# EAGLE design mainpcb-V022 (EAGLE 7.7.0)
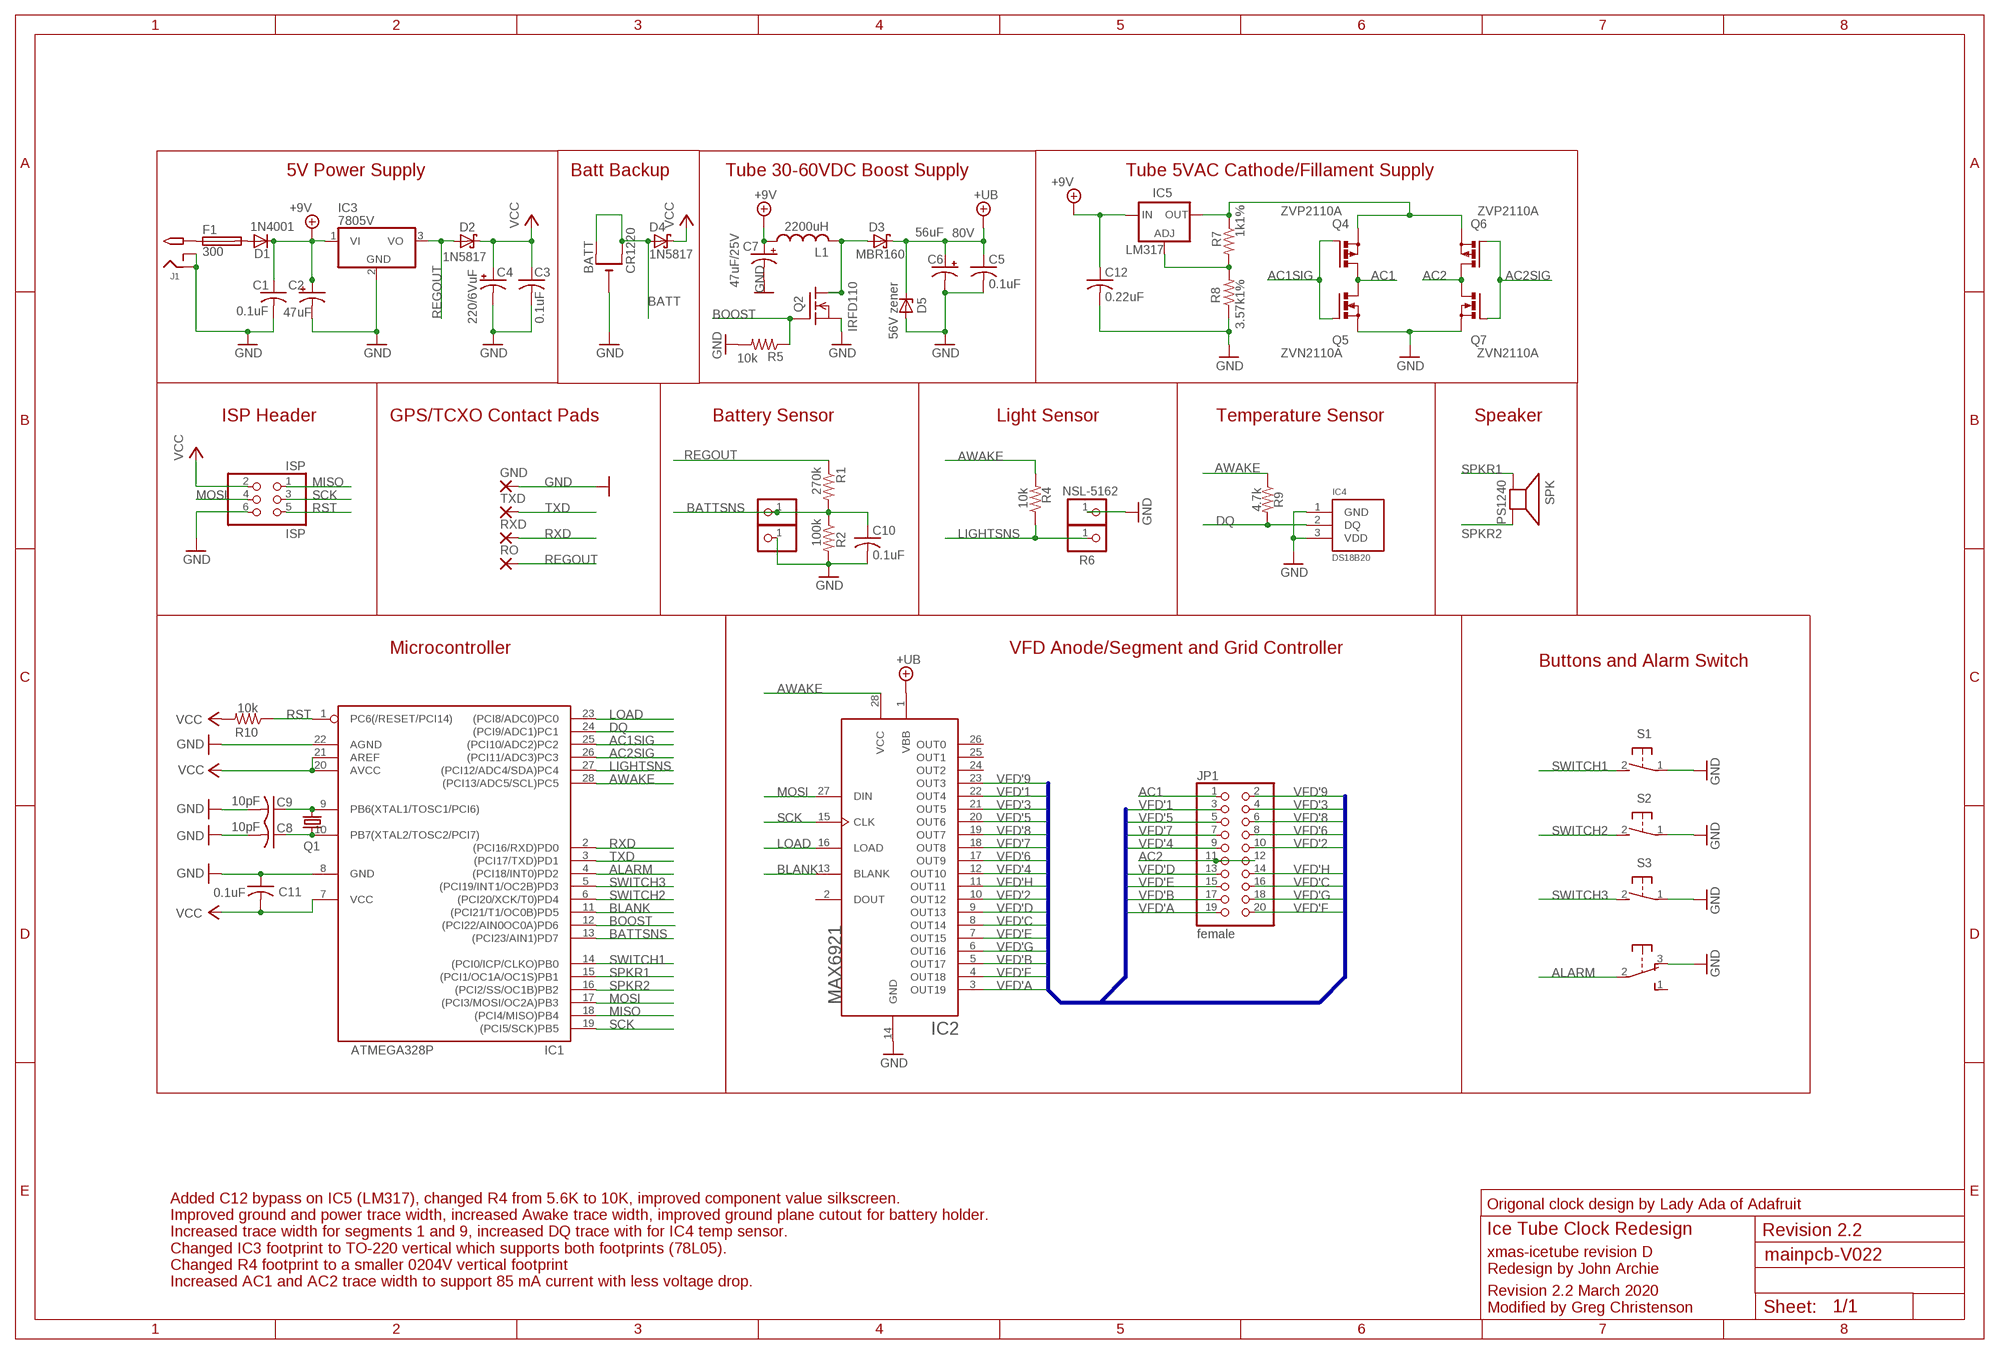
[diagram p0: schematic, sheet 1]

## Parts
BATT  CR1220  CR1220THM  [CR1220-THM]
C1  0.1uF  C-US025-025X050  [C025-025X050]
C2  47uF  CPOL-USE2.5-6  [E2,5-6]
C3  0.1uF  C-US025-025X050  [C025-025X050]
C4  220/6VuF  CPOL-USE2.5-6  [E2,5-6]
C5  0.1uF  C-US025-024X044  [C025-024X044]
C6  56uF  CPOL-USE3.5-8  [E3,5-8]
C7  47uF/25V  CPOL-USE2.5-6  [E2,5-6]
C8  10pF  C-US025-024X044  [C025-024X044]
C9  10pF  C-US025-024X044  [C025-024X044]
C10  0.1uF  C-US025-024X044  [C025-024X044]
C11  0.1uF  C-US025-025X050  [C025-025X050]
C12  0.22uF  C-US025-024X044  [C025-024X044]
CT2  PINHD-1X1  [1X01]
CT3  PINHD-1X1  [1X01]
D1  1N4001  1N4004  [DO41-10]
D2  1N5817  SCHOTTKY-DIODEDO41  [DO41-10]
D3  MBR160  SCHOTTKY-DIODEDO41  [DO41-10]
D4  1N5817  SCHOTTKY-DIODEDO41  [DO41-10]
D5  56V zener  ZENER-DIODEDO41Z10  [DO41Z10]
F1  300  FUSETE5  [TE5]
GND  1,6/0,9  [1,6/0,9]
IC1  ATMEGA328P  ATMEGA168PROUND  [DIL28/3]
IC2  MAX6921  [PLCC-S28]
IC3  7805V  7805TV  [TO220V]
IC4  DS18B20  [TO92]
IC5  LM317  [TO92-LINE]
ISP  ISP  PINHD-2X3  [2X03]
J1  2.1MMJACK  [PJ-102A]
JP1  female  PINHD-2X10  [2X10]
L1  2200uH  L  [6000]
Q1  32.768khz  CRYTALTC26V  [TC26V]
Q2  IRFD110  [DIL04]
Q4  ZVP2110A  [TO92-FLAT]
Q5  ZVN2110A  [TO92-FLAT]
Q6  ZVP2110A  [TO92-FLAT]
Q7  ZVN2110A  [TO92-FLAT]
R1  270k  R-US_0207/10  [0207/10]
R2  100k  R-US_0207/10  [0207/10]
R4  10k  R-US_0204/2V  [0204V]
R5  10k  R-US_0207/5V  [0207/5V]
R6  NSL-5162  PINHD-1X1  [1X01]
R6.1  PINHD-1X1  [1X01]
R7  1k1%  R-US_0207/5V  [0207/5V]
R8  3.57k1%  R-US_0207/5V  [0207/5V]
R9  4.7k  R-US_0207/10  [0207/10]
R10  10k  R-US_0207/5V  [0207/5V]
RO  1,6/0,9  [1,6/0,9]
RXD  1,6/0,9  [1,6/0,9]
S1  31-XX  [B3F-31XX]
S2  31-XX  [B3F-31XX]
S3  31-XX  [B3F-31XX]
SPK  PS1240  SPEAKER/PS12  [PS12]
SW1  OS102011MA1Q  [OS102011MA1Q]
TXD  1,6/0,9  [1,6/0,9]

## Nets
+9V: C1.1 C2.+ C7.+ C12.1 D1.C IC3.1(VI) IC5.3(IN) L1.1
+UB: C5.1 C6.+ D3.C D5.C IC2.1(VBB)
AC1: JP1.1 Q4.3(D) Q5.3(D)
AC1SIG: IC1.25((PCI10/ADC2)PC2) Q4.2(G) Q5.2(G)
AC2: JP1.11 JP1.12 Q6.3(D) Q7.3(D)
AC2SIG: IC1.26((PCI11/ADC3)PC3) Q6.2(G) Q7.2(G)
ALARM: IC1.4((PCI18/INT0)PD2) SW1.2(P)
AWAKE: IC1.28((PCI13/ADC5/SCL)PC5) IC2.28(VCC) R4.2 R9.1
BATT: BATT.+1(+) BATT.+2(+1) D4.A
BATTSNS: C10.1 CT2.1 IC1.13((PCI23/AIN1)PD7) R1.2 R2.1
BLANK: IC1.11((PCI21/T1/OC0B)PD5) IC2.13(BLANK)
BOOST: IC1.12((PCI22/AIN0OC0A)PD6) Q2.3(G) R5.1
DQ: IC1.24((PCI9/ADC1)PC1) IC4.2(DQ) R9.2
GND: BATT.- C1.2 C2.- C3.2 C4.- C5.2 C6.- C7.- C8.2 C9.2 C10.2 C11.1 C12.2 CT3.1 D5.A GND.1(P) IC1.8(GND) IC1.22(AGND) IC2.14(GND) IC3.2(GND) IC4.1(GND) IC4.3(VDD) ISP.6 J1.RING J1.RING_SW Q2.4(S) Q5.1(S) Q7.1(S) R2.2 R5.2 R6.1 R8.1 S1.1(P) S2.1(P) S3.1(P) SW1.3(O)
LIGHTSNS: IC1.27((PCI12/ADC4/SDA)PC4) R4.1 R6.1.1
LOAD: IC1.23((PCI8/ADC0)PC0) IC2.16(LOAD)
MISO: IC1.18((PCI4/MISO)PB4) ISP.1
MOSI: IC1.17((PCI3/MOSI/OC2A)PB3) IC2.27(DIN) ISP.4
N$1: C9.1 IC1.9(PB6(XTAL1/TOSC1/PCI6)) Q1.2
N$2: D3.A L1.2 Q2.1(D) Q2.2(D1)
N$3: C8.1 IC1.10(PB7(XTAL2/TOSC2/PCI7)) Q1.1
N$4: F1.1 J1.TIP
N$5: D1.A F1.2
N$6: IC5.1(ADJ) R7.2 R8.2
N$14: IC5.2(OUT) Q4.1(S) Q6.1(S) R7.1
REGOUT: D2.A IC3.3(VO) R1.1 RO.1(P)
RST: IC1.1(PC6(/RESET/PCI14)) ISP.5 R10.1
RXD: IC1.2((PCI16/RXD)PD0) RXD.1(P)
SCK: IC1.19((PCI5/SCK)PB5) IC2.15(CLK) ISP.3
SPKR1: IC1.15((PCI1/OC1A/OC1S)PB1) SPK.P$1(+)
SPKR2: IC1.16((PCI2/SS/OC1B)PB2) SPK.P$2(-)
SWITCH1: IC1.14((PCI0/ICP/CLKO)PB0) S1.2(S)
SWITCH2: IC1.6((PCI20/XCK/T0)PD4) S2.2(S)
SWITCH3: IC1.5((PCI19/INT1/OC2B)PD3) S3.2(S)
TXD: IC1.3((PCI17/TXD)PD1) TXD.1(P)
VCC: C3.1 C4.+ C11.2 D2.C D4.C IC1.7(VCC) IC1.20(AVCC) IC1.21(AREF) ISP.2 R10.2
VFD'1: IC2.22(OUT4) JP1.3
VFD'2: IC2.10(OUT12) JP1.10
VFD'3: IC2.21(OUT5) JP1.4
VFD'4: IC2.12(OUT10) JP1.9
VFD'5: IC2.20(OUT6) JP1.5
VFD'6: IC2.17(OUT9) JP1.8
VFD'7: IC2.18(OUT8) JP1.7
VFD'8: IC2.19(OUT7) JP1.6
VFD'9: IC2.23(OUT3) JP1.2
VFD'A: IC2.3(OUT19) JP1.19
VFD'B: IC2.5(OUT17) JP1.17
VFD'C: IC2.8(OUT14) JP1.16
VFD'D: IC2.9(OUT13) JP1.13
VFD'E: IC2.7(OUT15) JP1.15
VFD'F: IC2.4(OUT18) JP1.20
VFD'G: IC2.6(OUT16) JP1.18
VFD'H: IC2.11(OUT11) JP1.14
Unconnected: IC2.2(DOUT) IC2.24(OUT2) IC2.25(OUT1) IC2.26(OUT0) SW1.1(S) SW1.MT1(MT) SW1.MT2(MT)

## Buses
VFD'[1..9],VFD'_A,VFD'_B,VFD'_C,VFD'_D,VFD'_E,VFD'_F,VFD'_G,VFD'_H

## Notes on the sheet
- 5V Power Supply | Batt Backup | Tube 30-60VDC Boost Supply | Tube 5VAC Cathode/Fillament Supply
- 80V
- ISP Header | GPS/TCXO Contact Pads | Battery Sensor | Light Sensor | Temperature Sensor | Speaker
- Microcontroller | VFD Anode/Segment and Grid Controller
- Buttons and Alarm Switch
- Origonal clock design by Lady Ada of Adafruit
- Ice Tube Clock Redesign | Revision 2.2
- xmas-icetube revision D
- Redesign by John Archie
- Added C12 bypass on IC5 (LM317), changed R4 from 5.6K to 10K, improved component value silkscreen.
  Improved ground and power trace width, increased Awake trace width, improved ground plane cutout for battery holder.
  Increased trace width for segments 1 and 9, increased DQ trace with for IC4 temp sensor.
  Changed IC3 footprint to TO-220 vertical which supports both footprints (78L05).
  Changed R4 footprint to a smaller 0204V vertical footprint
  Increased AC1 and AC2 trace width to support 85 mA current with less voltage drop.
- Revision 2.2 March 2020
- Modified by Greg Christenson

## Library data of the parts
BATT = vfd:CR1220
C1 C3 C11 = minimidi:C-US: CAPACITOR, American symbol
C2 C4 C7 = minimidi:CPOL-US: POLARIZED CAPACITOR, American symbol
C5 C10 C12 = rcl-ez:C-US: CAPACITOR, American symbol
C6 = rcl-ez:CPOL-US: POLARIZED CAPACITOR, American symbol
C8 C9 = resistor:C-US: CAPACITOR, American symbol
CT2 CT3 R6 R6.1 = ybox2:PINHD-1X1: PIN HEADER
D1 = minimidi:1N4004: DIODE
D2-D4 = usbbuck:SCHOTTKY-DIODE: Schottky Diode
D5 = diode:ZENER-DIODE: Z-Diode
F1 = fuse:FUSE: Fuse
GND RO RXD TXD = wirepad:1,6/0,9: THROUGH-HOLE PAD
IC1 = avr:ATMEGA168*P: MICROCONTROLLER 16 kBytes FLASH 1 kBytes SRAM 512 Bytes EEPROM USART 8-channel 10 bit ADC
IC2 = vfd:MAX6921
IC3 = linear:78*: Positive VOLTAGE REGULATOR Source: http://cache.national.com/ds/LM/LM78L05.pdf http://www.fairchildsemi.com/ds/LM/LM7805.pdf
IC4 = jarchie:DS18B20
IC5 = jarchie:LM317: VOLTAGE REGULATOR
ISP = pinhead-ez:PINHD-2X3: PIN HEADER
J1 = minimidi:2.1MMJACK
JP1 = pinhead:PINHD-2X10: PIN HEADER
L1 = usbbuck:L
Q1 = crystal:CRYTAL: CRYSTAL
Q2 = vfd:IRFD110
Q4 Q6 = jarchie:ZVP2110A
Q5 Q7 = jarchie:ZVN2110A
R1 R2 R4 R5 R7-R10 = minimidi:R-US_: RESISTOR, American symbol
S1-S3 = switch-omron:31-XX: OMRON SWITCH
SPK = ybox2:SPEAKER: SPEAKER
SW1 = adaprog:OS102011MA1Q

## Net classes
0 default: clearance 0.205 mm

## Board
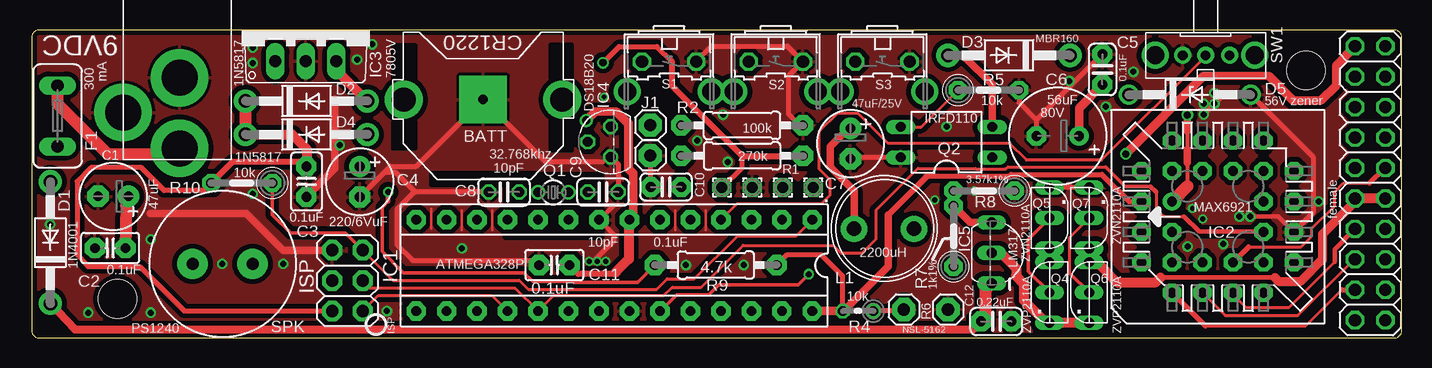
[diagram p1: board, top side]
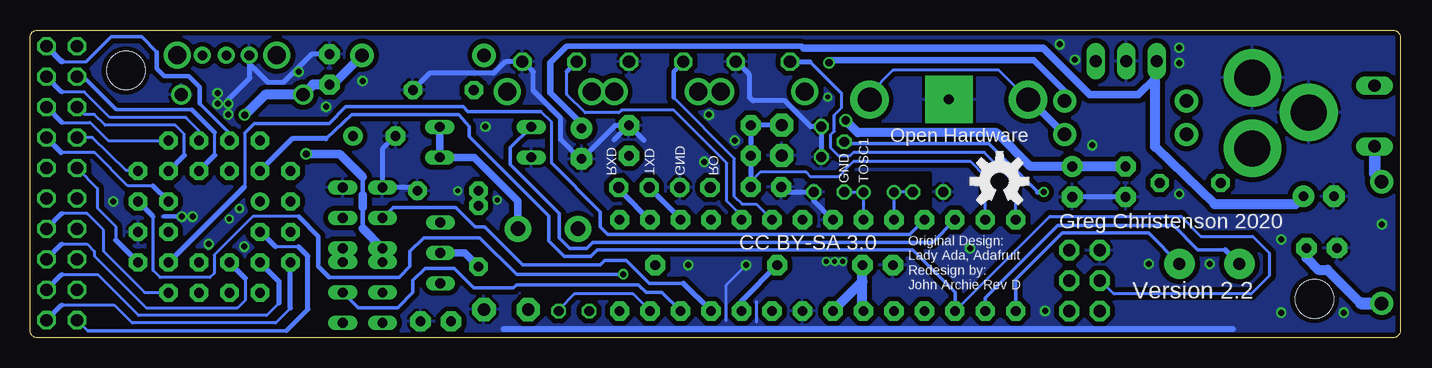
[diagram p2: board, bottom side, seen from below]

Size 114.2 x 25.71 mm. Coordinates in mm from the lower left corner, seen from the top.
Outline: 0,25.07 0,0.64 arc90 0.64,0 113.56,0 arc90 114.2,0.64 114.2,25.07 arc90 113.56,25.71 0.64,25.71 arc90 0,25.07
Copper layers (1*16): Top 0.0356mm / dielectric 1.5011mm / Bottom 0.0356mm
Design rules "LaenPCBOrder *": minimum track width 6mil, minimum drill 13mil, track to track 10mil, track to pad 10mil, pad to pad 10mil, via to via 10mil, smd to smd 6mil, copper to edge 15mil, drill to drill 8mil, minimum pad ring 7mil, minimum via ring 7mil, stop-mask expansion 4mil, vias tented up to drill 20mil, thermal gap 10mil
Holes 3.2 mm at 106.21,22.31 7.15,3.26

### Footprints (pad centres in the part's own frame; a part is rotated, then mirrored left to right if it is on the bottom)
CR1220-THM = drill 2 pad 3.175: +1 -6.604,0; +2 6.604,0 | drill 0.8 pad 3.962 square: - 0,0
C025-025X050 = drill 0.813 pad 1.676 octagon: 1 -1.27,0; 2 1.27,0
E2,5-6 = drill 0.813 pad 1.778: + -1.27,0 | drill 0.813 pad 1.778 octagon: - 1.27,0
C025-024X044 = drill 0.813 pad 1.676 octagon: 1 -1.27,0; 2 1.27,0
E3,5-8 = drill 0.813 pad 1.6: + -1.778,0 | drill 0.813 pad 1.6 octagon: - 1.778,0
C025-024X044' = drill 0.813 octagon: 1 -1.27,0; 2 1.27,0
1X01 = drill 1.016 pad 1.93 octagon: 1 0,0
DO41-10 = drill 1.118 pad 1.93: A 5.08,0; C -5.08,0
DO41Z10 = drill 1.118: A 5.08,0; C -5.08,0
TE5 = drill 1.016 long: 1 -2.54,0; 2 2.54,0
1,6/0,9 = drill 0.914 pad 1.6 octagon: 1 0,0
DIL28/3 = drill 0.813 pad 1.6 octagon: 1 -16.51,-3.81; 2 -13.97,-3.81; 3 -11.43,-3.81; 4 -8.89,-3.81; 5 -6.35,-3.81; 6 -3.81,-3.81; 7 -1.27,-3.81; 8 1.27,-3.81; 9 3.81,-3.81; 10 6.35,-3.81; 11 8.89,-3.81; 12 11.43,-3.81; 13 13.97,-3.81; 14 16.51,-3.81; 15 16.51,3.81; 16 13.97,3.81; 17 11.43,3.81; 18 8.89,3.81; 19 6.35,3.81; 20 3.81,3.81; 21 1.27,3.81; 22 -1.27,3.81; 23 -3.81,3.81; 24 -6.35,3.81; 25 -8.89,3.81; 26 -11.43,3.81; 27 -13.97,3.81; 28 -16.51,3.81
PLCC-S28 = drill 0.813 pad 1.524: 1 1.27,3.81 | drill 0.813 pad 1.524 octagon: 2 -1.27,6.35; 3 -1.27,3.81; 4 -3.81,6.35; 5 -6.35,3.81; 6 -3.81,3.81; 7 -6.35,1.27; 8 -3.81,1.27; 9 -6.35,-1.27; 10 -3.81,-1.27; 11 -6.35,-3.81; 12 -3.81,-6.35; 13 -3.81,-3.81; 14 -1.27,-6.35; 15 -1.27,-3.81; 16 1.27,-6.35; 17 1.27,-3.81; 18 3.81,-6.35; 19 6.35,-3.81; 20 3.81,-3.81; 21 6.35,-1.27; 22 3.81,-1.27; 23 6.35,1.27; 24 3.81,1.27; 25 6.35,3.81; 26 3.81,6.35; 27 3.81,3.81; 28 1.27,6.35
TO220V = drill 1.016 long: 1 -2.54,-2.54; 2 0,-2.54; 3 2.54,-2.54
TO92 = drill 0.813 octagon: 1 1.27,0; 2 0,1.905; 3 -1.27,0
TO92-LINE = drill 0.813 long: 1 -2.54,0; 2 0,0; 3 2.54,0
2X03 = drill 1.016 pad 1.676 octagon: 1 -2.54,-1.27; 2 -2.54,1.27; 3 0,-1.27; 4 0,1.27; 5 2.54,-1.27; 6 2.54,1.27
PJ-102A = drill 3 pad 4.8: RING 0.1,-3.39; RING_SW -4.6,-6.29; TIP 0.1,-9.29
2X10 = drill 1.016 octagon: 1 -11.43,-1.27; 2 -11.43,1.27; 3 -8.89,-1.27; 4 -8.89,1.27; 5 -6.35,-1.27; 6 -6.35,1.27; 7 -3.81,-1.27; 8 -3.81,1.27; 9 -1.27,-1.27; 10 -1.27,1.27; 11 1.27,-1.27; 12 1.27,1.27; 13 3.81,-1.27; 14 3.81,1.27; 15 6.35,-1.27; 16 6.35,1.27; 17 8.89,-1.27; 18 8.89,1.27; 19 11.43,-1.27; 20 11.43,1.27
6000 = drill 1.2 pad 2.184: 1 -2.5,0; 2 2.5,0
TC26V = drill 0.813: 1 -1.27,0; 2 1.27,0
DIL04 = drill 0.813 long: 1 -1.27,-3.81; 2 1.27,-3.81; 3 1.27,3.81; 4 -1.27,3.81
TO92-FLAT = drill 0.813 long: 1 -2.54,0; 2 0,0; 3 2.54,0
0207/10 = drill 0.813 pad 1.676 octagon: 1 -5.08,0; 2 5.08,0
0204V = drill 0.813 octagon: 1 -1.27,0; 2 1.27,0
0207/5V = drill 0.813 pad 1.524 octagon: 1 -2.54,0; 2 2.54,0
B3F-31XX = drill 1.016 octagon: 1 -2.261,-1.245; 2 2.261,-1.245 | drill 1.499 pad 2.159: 3 -3.505,1.245; 4 3.505,1.245
PS12 = drill 1 pad 2.54: P$1 -2.5,0; P$2 2.5,0
OS102011MA1Q = drill 0.8 pad 1.422: 1 -2,0; 2 0,0; 3 1.9,0 | drill 1.5 pad 2.184: MT1 -4.1,0; MT2 4.2,0

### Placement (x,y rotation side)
BATT  37.63,19.9 0 top
C1  6.55,7.51 180 top
C2  6.81,11.82 180 top
C3  22.9,13.04 270 top
C4  27.35,13.04 270 top
C5  89.24,22.41 90 top
C6  85.51,16.85 180 top
C7  68.24,16.22 270 top
C8  10pF  [C025-024X044']  39.36,12.18 180 top
C9  10pF  [C025-024X044']  47.62,12.18 0 top
C10  52.87,12.6 180 top
C11  43.56,6.08 0 top
C12  80.39,1.38 0 top
CT2  51.56,17.77 0 top
CT3  51.56,15.23 0 top
D1  1.57,7.96 90 top
D2  22.9,19.77 0 top
D3  81.45,23.58 180 top
D4  22.9,16.98 0 top
D5  96.52,20.31 0 top
F1  2.15,18.53 270 top
GND  60.07,12.56 0 top
IC1  48.56,6.06 180 top
IC2  98.85,10.12 90 top
IC3  22.86,25.64 0 top
IC4  48.25,16.37 90 top
IC5  80.01,7.1 270 top
ISP  26.33,4.79 90 top
J1  12.23,25.11 0 top
JP1  111.55,12.92 270 top
L1  71.04,9.11 0 top
Q1  43.48,12.15 0 top
Q2  76.24,16.35 90 top
Q4  84.83,3.8 90 top
Q5  84.83,10.02 270 top
Q6  88.13,3.8 90 top
Q7  88.13,10.02 270 top
R1  59.21,15.2 180 top
R2  59.21,17.74 0 top
R4  68.88,2.25 180 top
R5  79.75,20.69 0 top
R6  76.37,2.38 0 top
R6.1  72.69,2.38 0 top
R7  76.83,8.5 90 top
R8  79.37,12.28 180 top
R9  57.02,6.08 180 top
R10  17.52,12.94 180 top
RO  57.53,12.56 0 top
RXD  65.15,12.56 0 top
S1  53.13,21.81 180 top
S2  62.02,21.81 180 top
S3  70.91,21.81 180 top
SPK  15.92,6.19 180 top
SW1  97.83,23.58 180 top
TXD  62.61,12.56 0 top
U$1  [OSHW-LOGO-M]  33.4,13.07 0 bottom

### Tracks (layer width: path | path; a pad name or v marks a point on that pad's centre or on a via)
+9V
  Top 0.406: 68.04,17.49 C7.+
  Top 0.61: L1.1 68.54,12.27 66.54,14.26 66.54,15.99 68.04,17.49
  Top 0.686: D1.C 3.6,0.72 78.46,0.72 C12.1
  Top 0.813: C12.1 79.12,1.51
  Top 1.016: C2.+ 8.08,11.24 7.87,11.04 C1.1 | 79.12,1.51 79.5,1.89 79.5,4.05 IC5.3
  Bottom 0.406: 49.7,24.17 49.88,24.35 | 20.36,15.91 20.44,15.96 | IC3.1 20.44,23.1 20.44,22.85
  Bottom 0.457: 49.88,24.35 69.49,24.35 70.86,22.97
  Bottom 0.559: 70.86,22.97 70.86,20.49 68.24,17.87
  Bottom 0.61: 49.7,24.17 29.76,24.17 25.9,20.31 21.84,20.31 20.44,21.7 | 68.24,17.87 C7.+
  Bottom 0.711: 15.49,11.16 20.36,15.91
  Bottom 0.813: 20.44,15.96 20.44,21.7 20.44,22.85 | 15.49,11.16 8.74,11.16 C2.+ | C1.1 7.82,6.67 6.85,5.7 6.09,5.7 3.3,2.91 | 1.59,2.91 D1.C
  Bottom 1.016: 1.52,2.93 D1.C | 3.3,2.91 1.59,2.91
+UB  (via drill 0.6)
  Top 0.33: 96.31,17.26 96.31,15.71 | 96.31,14.64 96.31,12.67
  Top 0.61: v96.31,18.61 96.31,17.26 | 96.31,15.71 96.31,14.64
  Top 0.711: C5.1 87.29,19.2 C6.+
  Top 1.016: 96.31,12.67 IC2.1
  Bottom 0.406: 88.97,21.14 C5.1
  Bottom 0.711: D3.C 88.97,21.14
  Bottom 0.813: C5.1 90.6,21.14 D5.C 94.61,20.31 v96.31,18.61
AC1  (via drill 0.6)
  Top 0.508: JP1.1 110.28,24.29
  Top 0.61: Q4.3 Q5.3
  Top 0.686: 103.12,21.83 97.66,21.83
  Top 0.711: 110.28,24.29 108.71,22.72 108.71,21.07 107.44,19.8 105.15,19.8 103.12,21.83 | 97.66,21.83 v91.18,15.35
  Bottom 0.356: 86.48,13.45 86.48,11.93 | 86.48,10.91 86.48,9.13
  Bottom 0.711: v91.18,15.35 88.39,15.35 86.48,13.45 | 86.48,11.93 86.48,10.91 | 86.48,9.13 Q5.3
AC1SIG
  Top 0.305: Q5.2 83.05,8.24 83.05,5.58 Q4.2
  Bottom 0.305: Q5.2 83.94,10.91 78.73,10.91 77.08,9.26 76.32,9.26 73.15,6.08 66.67,6.08 66.29,6.46 64.51,6.46 62.61,4.56 59.76,4.56
  Bottom 0.406: IC1.25 59.76,4.56
AC2
  Top 0.381: 94.08,5.04 103.6,5.04
  Top 0.61: JP1.11 110.28,11.36 | Q7.3 Q6.3 88.77,6.34
  Top 0.762: 110.28,11.36 107.56,8.65 107.56,6.54 105.76,4.74 103.91,4.74 103.6,5.04
  Top 0.813: JP1.12 JP1.11 | 94.08,5.04 93.7,4.66 90.44,4.66 88.77,6.34
AC2SIG
  Top 0.254: Q7.2 86.48,8.37 86.48,5.45
  Top 0.305: 86.48,5.45 Q6.2
  Bottom 0.305: IC1.26 61.53,3.8 62.86,3.8 63.49,4.43 73.66,4.43 73.91,4.18 77.21,4.18 78.86,5.83 81.28,5.83 82.29,4.81 82.29,3.8 83.56,2.53 86.86,2.53 Q6.2
ALARM
  Top 0.254: IC1.4 58.79,11.21 65.83,11.21 66.54,11.93 66.54,13.2 65.65,14.08 65.65,17.26 67.18,18.78 68.83,18.78 71.37,16.24 81.53,16.24 82.93,14.85 89.15,14.85 97.83,23.53 SW1.2
AWAKE
  Top 0.254: 67.6,2.34 67.56,2.3 R4.2 | 74.54,13.45 74.62,13.5
  Top 0.406: IC2.28 91.46,11.39 89.2,13.65 81.63,13.65 81.45,13.5 74.62,13.5 | 67.56,2.3 67.56,5.19 65.78,6.97 62.99,6.97 R9.1 | 67.6,2.34 67.62,2.21
  Top 0.508: 71.37,10.27 74.54,13.45
  Top 0.61: 71.37,10.27 71.37,5.96 67.62,2.21
  Top 0.711: IC1.28 R4.2
BATT
  Bottom 0.254: BATT.+1 33.47,22.34 42.29,22.34 44.24,20.39
  Bottom 0.406: 30.9,19.9 BATT.+1 | BATT.+2 44.24,20.39 44.24,20.61
  Bottom 0.61: D4.A 30.9,19.9
BATTSNS
  Bottom 0.254: IC1.13 34.59,13.5 35.81,14.72 45.59,14.72 46.86,13.45 49.14,13.45 49.52,13.83 53.37,13.83 54.13,13.07 54.13,12.65
  Bottom 0.406: CT2.1 54.1,17.77 R2.1 R1.2 54.13,12.65 C10.1
BLANK
  Bottom 0.254: 96.31,17.08 96.31,12.64 | 39.67,9.85 IC1.11 | IC2.13 102.64,6.31 | 70.73,14.59 70.73,18.02 71.62,18.91 71.75,18.91
  Bottom 0.305: 96.31,17.08 95.5,17.89 89.28,17.89 87.88,19.29 78.1,19.29 77.72,18.91 71.75,18.91 | 39.67,9.85 40.89,8.62 66.04,8.62 66.67,9.26 66.67,10.53 70.73,14.59
  Bottom 0.406: 102.64,6.31 96.31,12.64
BOOST
  Top 0.254: Q2.3 74.14,17.62 R5.1
  Bottom 0.254: 37.13,9.85 IC1.12
  Bottom 0.305: Q2.3 74.16,15.88 74.16,14.47 70.1,10.4 70.1,8.37 69.21,7.48 67.81,7.48 67.31,7.99 38.98,7.99 37.13,9.85
DQ  (via drill 0.5)
  Top 0.305: R9.2 50.52,4.66 45.21,4.66 45.13,4.74 41.75,4.74 41.02,5.45 30.98,5.45 29.21,7.23 29.21,10.91 29.71,11.42
  Top 0.406: 29.71,11.42 v29.71,12.18
  Bottom 0.254: 46.1,16.37 IC4.2 45.97,16.24
  Bottom 0.305: 30.22,12.18 34.28,16.24 45.97,16.24
  Bottom 0.406: R9.2 54.91,3.12 IC1.24 | 30.22,12.18 v29.71,12.18
GND  (via drill 0.4, 0.5)
  Top 0.203: 53.64,10.66 53.64,9 | 56.18,10.66 56.18,9 | 33.32,10.78 33.32,9.13 | 35.86,10.66 35.86,9 | 38.4,10.66 38.4,9
  Top 0.356: IC1.8 48.51,8.65 | IC2.14 105.18,8.85 103.91,10.12 v101.54,10.12 | 47.26,9.81 48.49,11.04
  Top 0.406: IC2.14 106.8,10.46 106.8,15.1 D5.A 99.34,20.31 v97.69,18.66 | 37.53,19.8 BATT.- | BATT.- 42.82,14.72 47.62,14.72 IC4.3 48.89,14.47 C9.2 | 12.35,21.7 J1.RING | BATT.- 32.05,14.31 29.89,14.31 29.37,13.79 | C8.2 31.97,12.18 31.92,12.23 | C5.2 83.73,18.18 | R5.2 82.29,19.63 83.73,18.18 | CT3.1 51.56,12.62 C10.2 | S1.1 55.39,23.12 56.64,24.37 62.99,24.37 64.28,23.08 S2.1 63.11,21.89 63.11,18.66 64,17.77 64.26,17.77 R2.2 | C4.- 29.37,13.79 | 31.92,12.23 30.36,13.79 29.37,13.79 | C11.1 41.9,6.46 31.75,6.46 30.48,7.73 30.48,10.78 31.92,12.23 | 48.51,8.65 48.51,8.12 46.79,6.4 v46.46,6.4 | Q2.4 68.37,15.08 C7.- | 83.73,18.18 C6.- | Q7.1 Q5.1
  Top 0.61: ISP.6 20.98,7.33 17.9,10.4 9.9,10.4 | C3.2 25.27,14.14 25.27,19.93
  Bottom 0.254: 56.18,1.46 56.18,4.43 v54.53,6.08 | 53.64,1.33 53.64,3.04
  Bottom 0.356: 101.93,10.12 103.04,10.12
  Bottom 0.406: IC4.3 IC4.1 49.14,17.64 51.3,19.8 53.97,19.8 54.22,20.05 54.22,21.96 55.32,23.05 S1.1 | C5.2 90.73,23.68 93.09,21.32 94.36,21.32 95.93,22.9 SW1.3 95.88,23.53 95.88,21.7 97.69,19.9 v97.69,18.66 | 73.15,23.03 S3.1 | S3.1 74.59,23.05 75.56,22.09 80.89,22.09 R5.2 | J1.RING_SW 9.43,18.82 | IC1.8 48.89,11.47 C9.2 51.25,12.18 C10.2 | 63.04,16.5 R2.2 65.45,17.74 C7.- 68.37,14.95 69.97,16.55 69.97,18.35 72.26,20.64 72.26,22.21 73.1,23.05 S3.1 | C3.2 C4.- | C6.- 84.83,15.76 Q5.1 81.91,12.56 R8.1 | 64.28,17.79 65.53,16.55
  Bottom 0.508: 74.74,0.75 13.96,0.75
  other vias: 47.84,6.4 97.68,19.55 98.57,19.55 98.57,20.43 89.53,19.29 86.48,21.45 76.25,17.64 97.61,9.94 99.31,7.84 96.34,7.63 96.74,10.81 100.66,10.12 59.35,6.08 35.86,7.48 1.54,9.49 9.93,2.12 29.61,2.25 15.9,6.19 9.93,8.22 18.44,12.03 4.72,2.12 20.98,6.19 25.67,16.09 18.44,24.22 18.44,22.95 107.26,11.39 47.15,6.4 27.12,23.23 28.39,24.5 47.71,20.12 91.82,22.21 75.26,11.52 78.56,12.28 58.01,14.69 55.47,16.47 57.63,18.63
  pour Bottom (isolate 0.406, rank 2): -0.01,25.64 -0.01,-0.01 114.17,-0.01 114.17,25.64
  pour Top (isolate 0.406, rank 2): -0.01,25.64 -0.01,-0.01 114.17,-0.01 114.17,25.64
LIGHTSNS
  Top 0.406: R6.1.1 73.5,2.38 73.4,2.27 72.71,2.27 R4.1
  Bottom 0.254: IC1.27 63.95,3.67 68.83,3.67 70.15,2.35
  Bottom 0.406: 70.15,2.35 R4.1
LOAD  (via drill 0.5)
  Top 0.254: 52.42,2.25 IC1.23
  Top 0.305: 52.42,2.25 53.78,3.61 56.45,3.61 57.27,4.43 63.88,4.43 v64.77,5.32
  Bottom 0.254: 91.82,10.15 95.63,10.15 98.85,6.92 98.85,5.4 99.21,5.04 103.35,5.04 103.93,5.63 103.93,10.13
  Bottom 0.305: v64.77,5.32 73.66,5.32 76.7,8.37 81.4,8.37 82.55,7.23 82.55,5.96 83.43,5.07 89.28,5.07
  Bottom 0.356: 91.82,10.15 90.17,8.5 90.17,5.96 89.28,5.07
  Bottom 0.406: 103.93,10.13 IC2.16
MISO
  Top 0.254: IC1.18 39.64,2.25 38.35,3.54 28.9,3.54 ISP.1
MOSI
  Bottom 0.254: ISP.4 24.99,4.79 23.87,3.67 12.44,3.67 10.92,5.19 10.92,7.1 12.31,8.5 16.63,8.5 18.28,10.15 29.21,10.15 37.1,2.25 IC1.17 37.1,2.52
  Bottom 0.305: 89.53,16.62 87.37,18.66 78.48,18.66 77.59,17.64 77.59,16.8 70.99,10.2 70.99,8.12 69.67,6.79 67.48,6.79 66.92,7.35 40.63,7.35 37.1,3.82 37.1,2.52
  Bottom 0.406: 89.53,16.62 92.35,16.62 IC2.27
N$1
  Bottom 0.254: IC1.9 Q1.2 44.77,12.18 C9.1
N$2
  Top 0.406: 77.62,23.58 77.72,23.48
  Top 0.61: D3.A 77.62,23.58 | 77.72,23.48 80.05,21.17 Q2.2
  Bottom 0.406: 80.03,15.1 Q2.1
  Bottom 0.61: Q2.2 Q2.1 77.19,15.08 73.54,11.42 L1.2
N$3
  Bottom 0.254: IC1.10 Q1.1 42.18,12.18 C8.1
N$4
  Top 0.813: 11.87,15.35 J1.TIP
  Top 1.016: F1.1 2.15,19.55 6.34,15.35 11.87,15.35
N$5
  Bottom 0.965: F1.2 2.15,13.73 D1.A
N$6
  Top 0.61: R7.2 78.23,9.64 IC5.1
  Bottom 0.61: R8.2 R7.2
N$9
  cutout Top: 30.09,24.5 32,24.5 32,15.74 30.09,15.74
N$14
  Top 0.61: 84.2,1.64 84.58,1.51 Q4.1
  Top 0.813: Q6.1 Q4.1 | IC5.2 80.77,7.1 82.04,5.83 82.04,5.19 82.7,4.53 82.7,3.14 84.2,1.64
  Bottom 0.61: R7.1 77.97,7.1 IC5.2
N$18
  cutout Bottom: 39.24,8.24 39.24,13.7 47.75,13.7 47.75,8.24
N$19
  cutout Top: 39.49,13.7 47.49,13.7 47.49,8.37 39.49,8.37
N$21
  cutout Top: 33.27,13.83 42.29,13.83 42.29,12.69 33.27,12.69
N$23
  cutout Top: 43.17,24.5 43.17,15.61 45.08,15.61 45.08,24.5
REGOUT  (via drill 0.6)
  Top 0.406: v47.62,22.97 48.97,24.32 52.12,24.32 53.34,23.1 | RO.1 59.2,14.24 59.2,15.2
  Top 0.508: R1.1 59.2,15.2 53.34,21.07 53.34,23.1
  Top 0.813: D2.A 25.39,22.36 IC3.3
  Bottom 0.559: D2.A 27.98,20.61 30.55,23.18 47.42,23.18 v47.62,22.97
RST
  Top 0.254: IC1.1 63.69,8.5 58.8,8.5 55.24,4.94 52.95,4.94 52.09,4.08 41.37,4.08 40.63,4.81 30.12,4.81 ISP.5 27.58,7.33
  Top 0.305: 27.58,7.33 26.16,8.75 21.59,8.75 20.06,10.27 R10.1
RXD
  Bottom 0.305: IC1.2 62.58,9.87 | 64.77,12.05 RXD.1
  Bottom 0.406: 62.58,9.87 64.77,12.05
SCK
  Top 0.254: 93.72,12.18 93.72,10.78 94.36,10.15 96.03,10.15 | ISP.3 28.21,4.18 40.28,4.18 IC1.19 43.5,3.54 52.7,3.54 53.4,4.24 55.81,4.24 59.3,7.73 66.8,7.73 67.43,7.1 69.21,7.1 70.35,8.24 70.35,10.66 73.86,14.16 78.66,14.16 78.73,14.08 81.17,14.08 81.38,14.29 89.53,14.29 | 102.61,8.88 IC2.15
  Top 0.305: 93.24,12.66 91.16,12.66 89.53,14.29
  Top 0.356: 93.24,12.66 93.72,12.18 | 96.03,10.15 97.3,8.88 102.61,8.88
SPKR1
  Bottom 0.305: IC1.15 32.05,4.89 28.19,8.75 20.98,8.75 SPK.P$1
SPKR2
  Bottom 0.305: IC1.16 34.59,3.37 28.57,9.39 18.9,9.39 16.87,7.35 14.6,7.35
  Bottom 0.406: SPK.P$2 14.6,7.35
SWITCH1
  Bottom 0.254: IC1.14 32.05,12.86 34.67,15.48 45.59,15.48 45.87,15.2 46.81,15.2 47.49,15.89 47.49,16.93 47.16,17.26 47.16,18.58 46.6,19.16 46.6,20.43
  Bottom 0.305: 49.22,23.05 46.6,20.43
  Bottom 0.406: S1.2 49.22,23.05
SWITCH2
  Bottom 0.254: IC1.6 53.66,11.16 54.86,11.16 55.49,11.8 55.49,14.97 60.57,20.05
  Bottom 0.356: 60.57,20.05 60.57,22.23 S2.2
SWITCH3
  Bottom 0.254: IC1.5 54.91,10.19 56.13,11.42 56.13,14.59 60.57,19.04 64.89,19.04 65.14,18.79 67.93,18.79 69.46,20.32 69.46,22.23
  Bottom 0.356: S3.2 69.46,22.23
TXD
  Bottom 0.305: IC1.3 60.17,10.12 | 62.48,12.43 TXD.1
  Bottom 0.406: 60.17,10.12 62.48,12.43
VCC  (via drill 0.7)
  Top 0.406: ISP.2 12.72,2.25 9.01,5.96 4.69,5.96 3.81,6.97 3.81,13.07 4.95,14.21 9.14,14.21 11.04,12.31 14.35,12.31 R10.2 | C3.1 22.9,14.33 | 49.78,9.89 49.8,9.87 IC1.7
  Top 0.508: C11.2 45.56,5.35 48.53,5.35 48.69,5.5 | R10.2 16.75,14.71 22.52,14.71 22.9,14.33
  Top 0.711: 50.13,13.73 50.13,10.23 IC1.7 | v46.22,18.15 46.98,18.91 48.71,18.91 49.73,17.89
  Top 0.762: 49.73,17.89 49.73,14.14 50.13,13.73
  Top 0.813: 49.78,9.89 49.78,6.59 48.69,5.5 | D4.C 21.71,16.98 22.92,15.77 C3.1
  Top 1.016: D2.C D4.C
  Bottom 0.406: IC1.20 44.83,2.33
  Bottom 0.711: 44.83,4.71 C11.2
  Bottom 0.762: v46.22,18.15 45.21,17.13 33.65,17.13 30.83,14.31 C4.+
  Bottom 0.813: C3.1 C4.+ | 44.83,2.33 C11.2 | IC1.21 44.83,4.71
VFD'1
  Bottom 0.254: 110.21,21.81 JP1.3 | 98.8,15.25 98.8,17.13
  Bottom 0.305: 100.73,19.06 107.01,19.06
  Bottom 0.33: 107.01,19.06 109.75,21.81
  Bottom 0.356: 98.8,17.13 100.73,19.06
  Bottom 0.406: 109.75,21.81 JP1.3 | IC2.22 98.8,15.25
VFD'2
  Top 0.254: 101.41,7.61 105.79,7.61 106.68,8.5 106.68,9.13 108.58,11.04 108.58,12.18 109.32,12.92 111.48,12.92 | 112.75,14.19 JP1.10
  Top 0.406: IC2.10 101.41,7.61 | 111.48,12.92 112.75,14.19
VFD'3
  Bottom 0.254: IC2.21 100.12,17.31 101.21,18.4 107.54,18.4 109.67,20.54 111.55,20.54
  Bottom 0.406: 111.55,20.54 JP1.4
VFD'4
  Bottom 0.254: JP1.9 108.58,12.49 108.58,10.83 107.06,9.31 107.06,8.17
  Bottom 0.406: 107.06,8.17 IC2.12
VFD'5
  Bottom 0.254: IC2.20 102.66,13.91 | 101.34,15.23 101.34,17.01 102.1,17.77 107.95,17.77 108.83,18.66 109.67,18.66 JP1.5
  Bottom 0.406: 102.66,13.91 101.34,15.23
VFD'6
  Bottom 0.254: 103.95,12.69 106.04,12.69 108.81,15.46 111.6,15.46 | 112.82,16.67 JP1.8
  Bottom 0.406: IC2.17 103.95,12.69 | 111.6,15.46 112.82,16.67
VFD'7
  Bottom 0.254: IC2.18 105.22,13.96 106.17,13.96 109.01,16.73 JP1.7
VFD'8
  Bottom 0.254: 111.55,18 109.19,18 107.67,16.47 IC2.19
  Bottom 0.406: JP1.6 111.55,18
VFD'9
  Bottom 0.254: 111.55,23.08 109.49,23.08 | 97.53,16.52 IC2.23
  Bottom 0.305: 109.49,23.08 107.44,25.13 104.9,25.13 103.63,23.86 | 100.07,19.55 97.53,17.01
  Bottom 0.356: 103.63,23.86 103.63,22.47 102.99,21.83 100.96,21.83 100.07,20.94 100.07,19.55
  Bottom 0.406: 97.53,17.01 97.53,16.52
  Bottom 0.508: JP1.2 111.55,23.08
VFD'A
  Bottom 0.254: JP1.19 109.39,0.6 | 91.82,7.61 93.72,7.61 | 94.97,8.85 IC2.3
  Bottom 0.305: 92.86,0.6 109.39,0.6
  Bottom 0.356: 91.05,2.4 92.86,0.6
  Bottom 0.406: 91.05,2.4 91.05,6.85 91.82,7.61 | 93.72,7.61 94.97,8.85
VFD'B
  Top 0.254: 97.81,1 106.17,1 109.19,4.03
  Top 0.406: IC2.5 97.81,1 | 109.19,4.03 JP1.17
VFD'C
  Bottom 0.254: 111.55,7.84 109.44,7.84 108.83,7.23 108.83,6.85 104.52,2.53 96.9,2.53 96.26,3.16 96.26,5
  Bottom 0.406: JP1.16 111.55,7.84 | IC2.8 96.26,5
VFD'D
  Top 0.254: 108.58,6.34 104.77,2.53 101.21,2.53 100.12,3.62 IC2.9
  Top 0.356: JP1.13 108.58,7.41 108.58,6.34
VFD'E
  Top 0.254: IC2.7 99.46,1.89 105.53,1.89 110.21,6.57 JP1.15
VFD'F
  Bottom 0.254: 111.55,2.76 107.18,2.76 105.66,1.26 93.72,1.26 92.5,2.48
  Bottom 0.406: JP1.20 111.55,2.76 | 92.5,2.48 IC2.4
VFD'G
  Bottom 0.254: 111.55,5.3 108.56,5.3 105.15,1.89 94.48,1.89 93.47,2.91
  Bottom 0.406: JP1.18 111.55,5.3 | IC2.6 93.47,4.74 93.47,2.91
VFD'H
  Bottom 0.254: IC2.11 102.68,3.8 104.64,3.8 108.07,7.23 108.07,9 109.44,10.38 111.55,10.38
  Bottom 0.406: JP1.14 111.55,10.38

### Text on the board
tNames: 9VDC | mA | J1 | 80V | . | . | . | . | .
bNames: Open Hardware | TOSC1 | GND | Greg Christenson 2020 | CC BY-SA 3.0 | Original Design: / Lady Ada, Adafruit / Redesign by: / John Archie Rev D | Version 2.2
